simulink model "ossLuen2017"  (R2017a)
settings: Solver=VariableStepAuto  StartTime=0.0  StopTime=10.0  RelTol=1e-3
InitFcn:
  | initParams
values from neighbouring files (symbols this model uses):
  A = [-1 1 0 1;0 -8 0 1;0 0 -2 1; 0 0 0 -3]    [initParams.m]
  B = [1 0;0 0 ; 0 0; 0 1]    [initParams.m]
  C = eye(4)    [initParams.m]
  D = zeros(size(B))    [initParams.m]
  L = diag([10 20 30 30])    [initParams.m]
  x0 = [0.1;0;0.3]    [initParams.m]
  xs0 = [0;0;0;0]    [initParams.m]

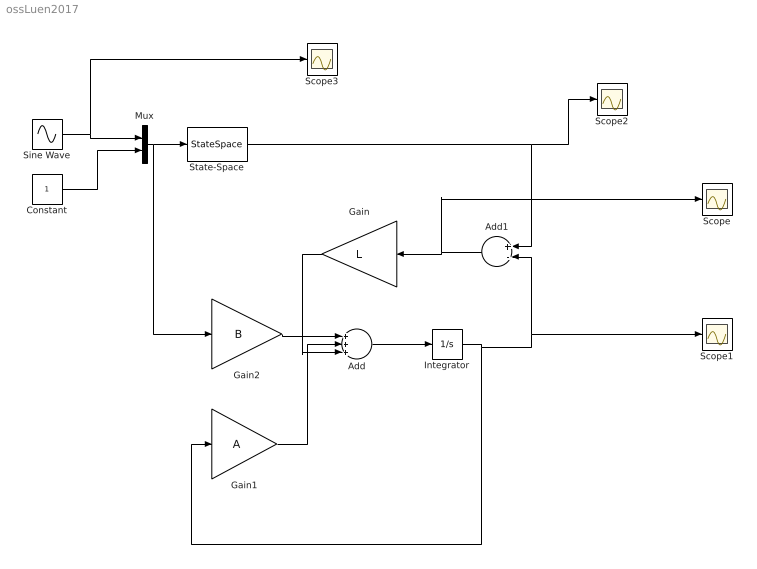
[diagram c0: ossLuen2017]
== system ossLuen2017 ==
  Add : Sum  Inputs=+++
  Add1 : Sum  Inputs=+-
  Constant : Constant
  Gain : Gain  Gain=L  Multiplication=Matrix(K*u) (u vector)
  Gain1 : Gain  Gain=A  Multiplication=Matrix(K*u) (u vector)
  Gain2 : Gain  Gain=B  Multiplication=Matrix(K*u) (u vector)
  Integrator : Integrator  InitialCondition=xs0
  Mux : Mux  Inputs=2
  Scope{,1..3} (4 alike) : Scope
  Sine Wave : Sin  SampleTime=0
  State-Space : StateSpace  A=A  B=B  C=C  D=D  X0=x0
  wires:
  Sine Wave/1 -> Scope3/1, Mux/1
  Constant/1 -> Mux/2
  Mux/1 -> Gain2/1, State-Space/1
  Gain2/1 -> Add/1
  Add/1 -> Integrator/1
  Integrator/1 -> Add1/2, Scope1/1, Gain1/1
  Gain1/1 -> Add/2
  Gain/1 -> Add/3
  Add1/1 -> Scope/1, Gain/1
  State-Space/1 -> Scope2/1, Add1/1
